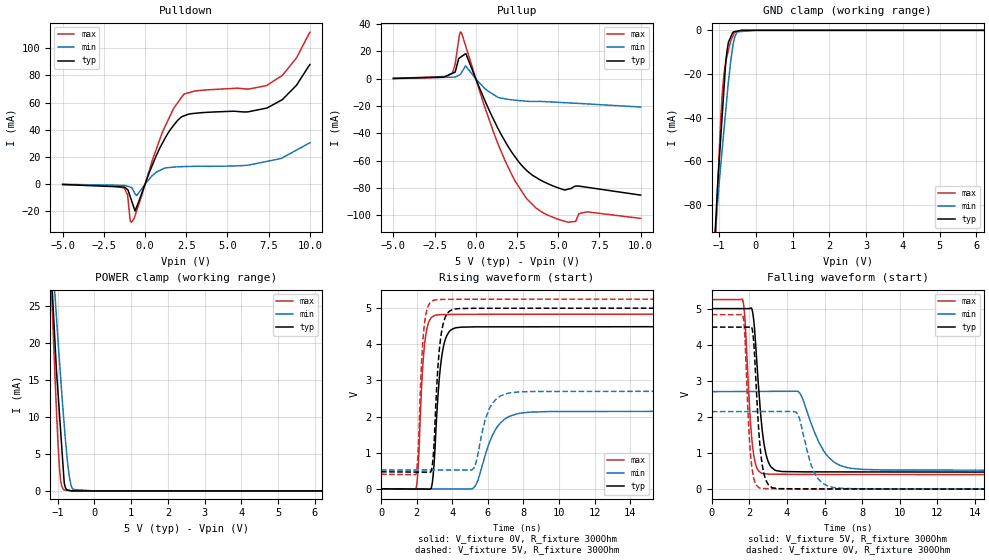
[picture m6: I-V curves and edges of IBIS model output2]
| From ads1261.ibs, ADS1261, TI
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|   output2 Model
[Model]   output2
Model_type   3-state
Polarity   Non-Inverting
Vmeas = 2.5
Vref = 0
Cref = 20pF
Rref = 100000
|   typ   min   max
C_comp   2.895pF   2.739pF   3.074pF
|  Where Nom  PVT is Nominal Process,   5V,  27C
|   Fast PVT is Strong Process,   5.25V, -40C
|   Slow PVT is Weak Process,   2.7V, 135C
[Voltage Range]   5   2.7   5.25
|Junction Temperature
[Temperature Range]   27   135   -40
[Pullup Reference]   5   2.7   5.25
[Pulldown Reference]   0   -0   0
[Power Clamp Reference]   5   2.7   5.25
[GND Clamp Reference]   0   0   0
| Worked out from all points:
|   slope of the pulldown table from 0 to 0.75 V, typ, clamps not added: 32.8 ohm
|   slope of the pullup table from 0 to 0.75 V, typ, clamps not added: 35 ohm
|   GND clamp passes 1 mA (typ) near -0.63 V on its own axis
|   POWER clamp passes 1 mA (typ) near -0.82 V on its own axis
|   falling waveform, V_fixture 5V, R_fixture 300Ohm: 20-80 % time 423ps typ, 1.11ns min, 324ps max; typ from 5 V to 0.47 V
|   rising waveform, V_fixture 0V, R_fixture 300Ohm: 20-80 % time 383ps typ, 972ps min, 296ps max; typ from 0 V to 4.49 V
|   rising waveform, V_fixture 5V, R_fixture 300Ohm: 20-80 % time 338ps typ, 696ps min, 267ps max; typ from 0.47 V to 5 V
|   falling waveform, V_fixture 0V, R_fixture 300Ohm: 20-80 % time 339ps typ, 705ps min, 271ps max; typ from 4.49 V to 0 V
[Pulldown]
|   Voltage   I(typ)   I(min)   I(max)
-5V       -193.4uA   -112.8uA   -189.4uA
-1.25V    -2.091mA   -817.1uA   -2.89mA
-1.054V   -4.073mA   -1.54mA    -8.17mA
-923.5mV  -8.295mA   -2.024mA   -24.5mA
-821.5mV  -11.96mA   -2.401mA   -27.9mA
-607.2mV  -19.66mA   -7.076mA   -23.2mA
1.019V    29.34mA    10.84mA    37.06mA
2.333V    50.07mA    12.93mA    65.78mA
7.362V    55.87mA    16.69mA    72.38mA
8.33V     62.16mA    19.38mA    79.94mA
9.187V    72.67mA    25.06mA    92.75mA
10V       87.97mA    30.44mA    111.7mA
[GND Clamp]
|   Voltage   I(typ)   I(min)   I(max)
-5V       -1.52A     -1.098A    -1.984A
-1.128V   -98.9mA    -97.61mA   -109.8mA
-1.036V   -69.42mA   -77.91mA   -70.48mA
-968.3mV  -52.25mA   -64.15mA   -44.78mA
-916.6mV  -39.09mA   -54.61mA   -29.21mA
-869.5mV  -27.12mA   -45.93mA   -20.2mA
-821.4mV  -14.89mA   -37.05mA   -14.67mA
-783.3mV  -9.118mA   -30.02mA   -11.7mA
-607.2mV  -696.4uA   -5.31mA    -1.885mA
-508.9mV  -378.5uA   -709.8uA   -614.5uA
-134.8uV  -255.3pA   0A         0A
10V       0A         0A         0A
[Pullup]
|   Voltage   I(typ)   I(min)   I(max)
-5V       265.3uA    145.7uA    281.3uA
-1.411V   4.079mA    1.21mA     4.301mA
-1.25V    4.943mA    1.258mA    10.87mA
-1.003V   15.14mA    2.711mA    31.38mA
-886.4mV  16.11mA    4.169mA    34.03mA
-607.2mV  18.45mA    9.28mA     23.71mA
1.34V     -36.22mA   -13.49mA   -47.4mA
2.248V    -54.85mA   -15.46mA   -71.74mA
3.115V    -67.4mA    -16.43mA   -88.13mA
5.606V    -80.74mA   -17.62mA   -104.9mA
6.757V    -79.39mA   -18.37mA   -97.35mA
10V       -85.11mA   -20.66mA   -102.1mA
[POWER Clamp]
|   Voltage   I(typ)   I(min)   I(max)
-5V       436.4mA    340.8mA    564.7mA
-1.16V    28.56mA    33.03mA    26.39mA
-1.131V   25.6mA     30.82mA    22.66mA
-1.087V   21.5mA     27.61mA    17.27mA
-1.036V   16.57mA    23.77mA    11.23mA
-952.6mV  10.59mA    17.71mA    3.27mA
-891.1mV  6.155mA    13.45mA    675.6uA
-821.5mV  1.14mA     8.971mA    135.8uA
-736.5mV  133.7uA    4.151mA    72.63uA
-684.6mV  80.66uA    2.005mA    34.08uA
-581.1mV  1.37uA     201.2uA    825.8nA
10V       0A         0A         0A
[Ramp]
R_load = 300
|   typ   min   max
dV/dt_r   2.69213/3.82354e-10   1.2877/9.69247e-10   2.89953/2.94922e-10
dV/dt_f   2.71779/4.22331e-10   1.30726/1.09923e-09   2.90858/3.22927e-10
[Falling Waveform]
V_fixture = 5V
V_fixture_min = 2.7V
V_fixture_max = 5.25V
R_fixture = 300Ohm
C_fixture = 0F
|   Time   V(typ)   V(min)   V(max)
0s        5V         2.7V       5.25V
1.656ns   4.999V     2.704V     5.229V
2.194ns   4.835V     2.705V     1.094V
2.641ns   1.855V     2.706V     443.5mV
2.933ns   873mV      2.707V     422.2mV
3.356ns   526.7mV    2.708V     414.5mV
4.686ns   481mV      2.66V      408.3mV
5.95ns    478.3mV    1.065V     406.7mV
7.237ns   477.6mV    593.4mV    406.3mV
20ns      470.3mV    520.9mV    402.4mV
[Rising Waveform]
V_fixture = 0V
V_fixture_min = 0V
V_fixture_max = 0V
R_fixture = 300Ohm
C_fixture = 0F
|   Time   V(typ)   V(min)   V(max)
0s        61.82uV    597.1uV    6.154uV
1.973ns   -6.339mV   -2.21mV    15.14mV
2.434ns   -7.836mV   -2.867mV   3.941V
2.962ns   581.5mV    -3.618mV   4.785V
3.415ns   3.681V     -4.263mV   4.821V
4.052ns   4.431V     -5.168mV   4.825V
5.3ns     4.481V     86.03mV    4.828V
6.433ns   4.481V     1.644V     4.829V
7.637ns   4.482V     2.076V     4.829V
20ns      4.487V     2.147V     4.833V
[Rising Waveform]
V_fixture = 5V
V_fixture_min = 2.7V
V_fixture_max = 5.25V
R_fixture = 300Ohm
C_fixture = 0F
|   Time   V(typ)   V(min)   V(max)
0s        470.3mV    520.9mV    402.4mV
1.973ns   463.2mV    520.7mV    417mV
2.391ns   461.7mV    520.7mV    4.337V
2.907ns   774.5mV    520.6mV    5.207V
3.356ns   4.202V     520.6mV    5.24V
3.982ns   4.952V     520.5mV    5.243V
5.224ns   4.995V     581.1mV    5.246V
6.088ns   4.995V     2.219V     5.246V
7.137ns   4.995V     2.645V     5.247V
20ns      5V         2.7V       5.25V
[Falling Waveform]
|Gnd
V_fixture = 0V
V_fixture_min = 0V
V_fixture_max = 0V
R_fixture = 300Ohm
C_fixture = 0F
|   Time   V(typ)   V(min)   V(max)
0s        4.487V     2.147V     4.833V
1.656ns   4.486V     2.149V     4.811V
2.01ns    4.49V      2.149V     1.335V
2.184ns   4.326V     2.149V     433.5mV
2.518ns   1.506V     2.15V      39.76mV
3.194ns   46.18mV    2.15V      12.01mV
4.496ns   10.01mV    2.13V      6.331mV
5.449ns   7.262mV    467.8mV    4.597mV
6.433ns   6.775mV    52.92mV    4.286mV
20ns      61.85uV    597.1uV    6.061uV
